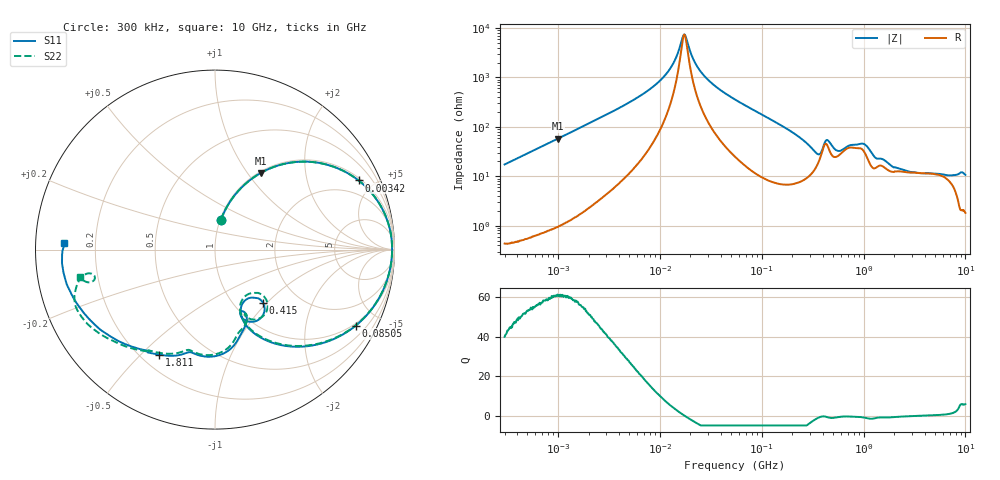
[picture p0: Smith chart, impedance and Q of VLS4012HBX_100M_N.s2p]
! S-Parameter Data Generated by TDK Corporation
! Copyright(C) 2023 TDK Corporation.
! All Rights Reserved.
! TDK P/N: VLS4012HBX-100M-N (Inductor)
! Property: L=10uH at 1MHz
! Size(LxWxT): 4x4x1.2mm
! Model Type: s2p (Touchstone File Format Version 1.0)
! Frequency: DC=Yes Start=0.3MHz Stop=10000MHz 802points Log-sweep
! Model Generated on June 16, 2023
! Port Assignments:
!  1 ---@@@--- 2
! Applicable Conditions:
!  Temperature = 25 degC
!  DC Bias Current = 0 A
!  Small Signal Operation
! Terms and conditions regarding TDK Simulation Models
! (1)This simulation model is being provided solely for informational purposes. Please refer to the specifications of the products in terms of detailed characteristics of such products.
! (2)In no event shall TDK Corporation of any of its subsidiaries be liable for any loss or damage arising, directly or indirectly,
!  From any information contained in this simulation model, including, but not limited to loss or damages arising from any inaccuracies, omissions or errors in connection with such information.
! (3)Any and all copyrights on this simulation model are owned by TDK Corporation.
!  Duplication or redistribution of this simulation model without prior written permission from TDK Corporation is prohibited.
! (4)This simulation model is subject to any modification or change without any prior notice.
! (5)Neither TDK Corporation nor any of its subsidiaries shall make any warranty, express or implied,
!  Including but not limited to the correctness, implied warranties of merchantability and fitness for a particular purpose with respect to this simulation models.
! (6)The use of this simulation model shall be deemed to have consented to the terms and conditions hereof.
# Hz S MA R 50
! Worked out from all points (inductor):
!   801 points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, 300 kHz to 10 GHz, reference 50 ohm
!   read as one part in series: L = 9.19 uH near 318.3 kHz
!   highest Q = 60.9 at 1.003 MHz (marker M1), where L = 9.21 uH
!   self-resonance near 17.41 MHz
!   S11 on the Smith chart (normalised r, x): 300 kHz: 1.01, +0.35; 3.42 MHz: 1.12, +4.09; 85.05 MHz: 0.91, -3.74; 415 MHz: 1.35, -0.94; 1.811 GHz: 0.27, -0.57; 10 GHz: 0.09, +0.02
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300000  0.1699 78.7  0.9812 -9.8  0.9812 -9.8  0.1698 78.8
1003308  0.4983 59.1  0.8588 -29.9  0.8589 -29.9  0.4983 59.1
1713600  0.6988 44.6  0.7027 -44.4  0.7028 -44.4  0.6988 44.6
3419615  0.8881 25.7  0.4364 -62.8  0.4366 -62.8  0.8881 25.7
9671944  0.981 6.5  0.1227 -78.1  0.1227 -78.1  0.9812 6.6
1.322782e7  0.9861 2.5  0.05616 -74.9  0.05619 -74.9  0.9862 2.5
1.740512e7  0.9866 -0.9  0.01328 -2.5  0.01328 -2.4  0.9868 -0.8
2.189307e7  0.9849 -3.7  0.04674 68.8  0.04677 68.8  0.985 -3.6
2.630692e7  0.9818 -6.0  0.08303 73.8  0.08306 73.8  0.982 -5.9
5.477226e7  0.9469 -18.0  0.2624 68.1  0.2624 68.1  0.9472 -17.8
8.505279e7  0.8909 -28.4  0.4084 58.6  0.4085 58.6  0.8911 -28.1
1.720721e8  0.6936 -51.2  0.6755 35.3  0.6756 35.3  0.6935 -50.7
3.126428e8  0.4139 -68.4  0.8188 8.1  0.819 8.1  0.4095 -68.3
3.730642e8  0.3284 -58.9  0.7814 -3.2  0.7816 -3.2  0.3107 -58.4
4.149731e8  0.3977 -47.9  0.6667 -5.7  0.6668 -5.7  0.3778 -43.7
5.497689e8  0.3867 -68.6  0.7394 -6.5  0.7396 -6.5  0.402 -65.4
9.216398e8  0.5219 -76.2  0.6236 -17.5  0.6238 -17.5  0.5051 -76.9
1.24442e9  0.5932 -100.0  0.6806 -22.3  0.6808 -22.3  0.5856 -100.3
1.767019e9  0.6581 -116.8  0.6225 -38.2  0.6227 -38.2  0.6489 -117.1
1.810952e9  0.6636 -118.1  0.6185 -39.3  0.6187 -39.4  0.6545 -118.5
4.457691e9  0.8161 -155.7  0.3643 -77.7  0.3644 -77.8  0.8158 -148.2
1e10  0.8429 177.6  0.2212 -110.7  0.2214 -110.9  0.7668 -168.4
